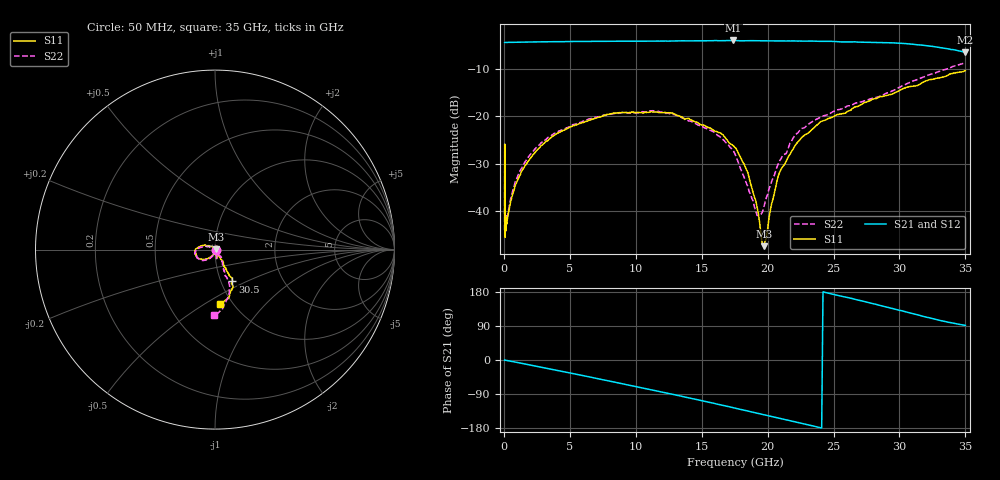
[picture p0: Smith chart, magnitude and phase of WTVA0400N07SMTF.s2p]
! 50 ohm 2-Port S-parameters measured by Modelithics Inc support@modelithics.com  Tampa, FL USA 813-866-6335 (February 2024)
! Smiths Interconnect,  4dB P/N: WTVA0400N07SMTF, Temperature: 25C
! Board: 10 mil Rogers 4350B, Mounting Pad Dimensions: Length: 15 mils, Width: 25 mils, Gap: 40 mils.
# Hz S MA R 50
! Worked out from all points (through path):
!   486 points, 50 MHz to 35 GHz, reference 50 ohm
!   highest |S21| = -3.95 dB at 17.4 GHz (marker M1); lowest = -6.5 dB at 35 GHz (marker M2)
!   group delay of S21, straight-line fit = 21.3 ps
!   lowest |S11| = -47.4 dB at 19.7 GHz (marker M3), VSWR 1.01, Z = 50.4 + j0.189 ohm
!   |S11| at or under -10 dB: start of sweep to end of sweep
!   |S22| runs from -45.3 to -8.7 dB; largest |S21 - S12| = 0.014
!   S11 on the Smith chart (normalised r, x): 50 MHz: 1.02, -0.01; 30.5 GHz: 1.13, -0.42; 35 GHz: 0.87, -0.58
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5e7  0.008971 -22.7  0.604 -0.4  0.6041 -0.3  0.006274 -13.3
8e7  0.008555 -32.6  0.6048 -0.4  0.6038 -0.5  0.007464 -16.8
9e7  0.005263 -31.9  0.6045 -0.5  0.6041 -0.5  0.005413 -31.9
1.1e8  0.006677 -30.8  0.6045 -0.7  0.6042 -0.7  0.006628 -34.2
5e8  0.01242 -79.8  0.6057 -3.1  0.6055 -3.1  0.01332 -81.6
9e8  0.01912 -95.7  0.6087 -5.7  0.6087 -5.6  0.02086 -95.8
2.25e9  0.03986 -115.8  0.6117 -15.0  0.6118 -14.9  0.04354 -113.4
3.95e9  0.0648 -129.3  0.6159 -26.8  0.6158 -26.8  0.06712 -126.9
5.9e9  0.08562 -140.6  0.6191 -40.5  0.6192 -40.4  0.08712 -136.2
1.17e10  0.1102 -176.4  0.6238 -82.6  0.6239 -82.5  0.1131 -171.8
1.58e10  0.07274 161.8  0.63 -113.2  0.6302 -113.2  0.06978 166.4
1.74e10  0.04892 154.0  0.6343 -126.0  0.6341 -125.9  0.0432 156.5
1.76e10  0.04589 151.6  0.6327 -127.9  0.6328 -127.6  0.03779 154.5
1.84e10  0.02714 138.6  0.63 -133.9  0.6299 -133.7  0.01949 169.5
1.92e10  0.01104 117.8  0.6284 -140.4  0.6285 -140.2  0.008997 -142.8
1.97e10  0.004251 26.2  0.6275 -144.2  0.6273 -143.9  0.01081 -87.1
2.1e10  0.02729 -58.1  0.6274 -154.4  0.6272 -154.2  0.03536 -54.1
2.22e10  0.05183 -58.8  0.625 -164.2  0.625 -163.8  0.06562 -55.9
2.34e10  0.07344 -56.3  0.6248 -173.7  0.6249 -173.4  0.08807 -61.9
2.92e10  0.1692 -60.5  0.6008 138.3  0.6008 138.9  0.179 -67.3
3.05e10  0.2021 -61.5  0.5868 126.8  0.587 127.6  0.2196 -68.4
3.5e10  0.3044 -84.8  0.4758 91.3  0.4755 91.7  0.3666 -90.4
